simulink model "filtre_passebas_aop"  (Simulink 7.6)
settings: Solver=ode45  StartTime=0.0  StopTime=10.0  RelTol=1e-3
libraries: fl_lib x8, elec_lib x2

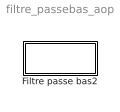
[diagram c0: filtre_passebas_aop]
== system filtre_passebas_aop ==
  Filtre passe bas2 : Subsystem

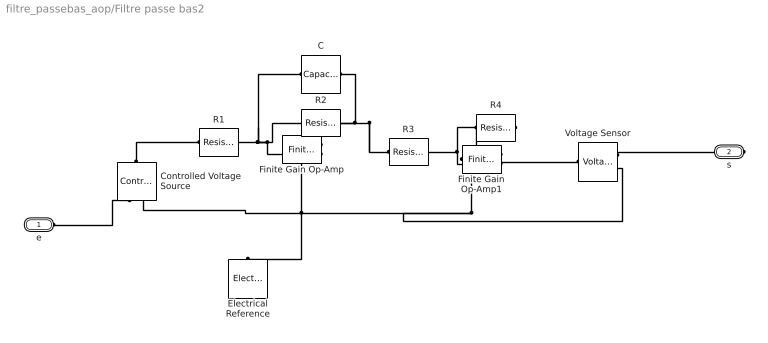
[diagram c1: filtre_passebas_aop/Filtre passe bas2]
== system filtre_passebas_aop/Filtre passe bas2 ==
  C : fl_lib/Electrical/Electrical Elements/Capacitor  DialogController=NetworkEngine.DynNeDlgSource  SystemSampleTime=-1  c=1e-3 F  v0=0 V  r=1e-6 Ohm  g=0 1/Ohm  i_Log=off  v_Log=off  vc_Log=off  LocalVarNames=|i|v|vc  LocalVarDescs=|i|v|Internal variable for voltage across capacitor term  LocalVarLogging=[0 0 0]
  Controlled Voltage Source : fl_lib/Electrical/Electrical Sources/Controlled Voltage Source  DialogController=NetworkEngine.DynNeDlgSource  SystemSampleTime=-1  i_Log=off  v_Log=off  LocalVarNames=|i|v  LocalVarDescs=|i|v  LocalVarLogging=[0 0]
  Electrical Reference : fl_lib/Electrical/Electrical Elements/Electrical Reference  DialogController=NetworkEngine.DynNeDlgSource  SystemSampleTime=-1  i_Log=off  LocalVarNames=|i  LocalVarDescs=|i  LocalVarLogging=0
  Finite Gain Op-Amp : elec_lib/Integrated Circuits/Finite Gain Op-Amp  DialogController=NetworkEngine.DynNeDlgSource  SystemSampleTime=-1  A=1000  Rin=1e+6 Ohm  Rout=100 Ohm  Vmin=-15 V  Vmax=15 V  LocalVarLogging=[]
  Finite Gain Op-Amp1 : elec_lib/Integrated Circuits/Finite Gain Op-Amp  DialogController=NetworkEngine.DynNeDlgSource  SystemSampleTime=-1  A=1000  Rin=1e+6 Ohm  Rout=100 Ohm  Vmin=-15 V  Vmax=15 V  LocalVarLogging=[]
  R1 : fl_lib/Electrical/Electrical Elements/Resistor  DialogController=NetworkEngine.DynNeDlgSource  SystemSampleTime=-1  R=1e3 Ohm  i_Log=off  v_Log=off  LocalVarNames=|i|v  LocalVarDescs=|i|v  LocalVarLogging=[0 0]
  R2 : fl_lib/Electrical/Electrical Elements/Resistor  DialogController=NetworkEngine.DynNeDlgSource  SystemSampleTime=-1  R=10e3 Ohm  i_Log=off  v_Log=off  LocalVarNames=|i|v  LocalVarDescs=|i|v  LocalVarLogging=[0 0]
  R3 : fl_lib/Electrical/Electrical Elements/Resistor  DialogController=NetworkEngine.DynNeDlgSource  SystemSampleTime=-1  R=10e3 Ohm  i_Log=off  v_Log=off  LocalVarNames=|i|v  LocalVarDescs=|i|v  LocalVarLogging=[0 0]
  R4 : fl_lib/Electrical/Electrical Elements/Resistor  DialogController=NetworkEngine.DynNeDlgSource  SystemSampleTime=-1  R=10e3 Ohm  i_Log=off  v_Log=off  LocalVarNames=|i|v  LocalVarDescs=|i|v  LocalVarLogging=[0 0]
  Voltage Sensor : fl_lib/Electrical/Electrical Sensors/Voltage Sensor  DialogController=NetworkEngine.DynNeDlgSource  SystemSampleTime=-1  i1_Log=off  v1_Log=off  LocalVarNames=|i1|v1  LocalVarDescs=|i1|v1  LocalVarLogging=[0 0]
  e : PMIOPort  Port=1  Side=Left
  s : PMIOPort  Port=2  Side=Right
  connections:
  Finite Gain Op-Amp/LConn2 -- R2/LConn1 -- C/LConn1 -- R1/RConn1
  C/RConn1 -- Finite Gain Op-Amp/RConn1 -- R3/LConn1 -- R2/RConn1
  Finite Gain Op-Amp/LConn1 -- Electrical Reference/LConn1 -- Controlled Voltage Source/RConn2 -- Finite Gain Op-Amp1/LConn1 -- Voltage Sensor/RConn2
  R4/LConn1 -- Finite Gain Op-Amp1/LConn2 -- R3/RConn1
  Finite Gain Op-Amp1/RConn1 -- R4/RConn1 -- Voltage Sensor/LConn1
  e/RConn1 -- Controlled Voltage Source/RConn1
  Controlled Voltage Source/LConn1 -- R1/LConn1
  Voltage Sensor/RConn1 -- s/RConn1
